| IBIS file stm32mp251_253_255_257_tfbga436.ibs
[IBIS ver] 5.1
[File name] stm32mp251_253_255_257_tfbga436.ibs
[File Rev] 1.3
[Date] 09-10-2025
[Source] Data Created at STMicroelectronics
[Notes]  File originated from ELDO simulations.
[Disclaimer]  This information is for modeling purpose only and is
   not guaranted. The information is subject to change without
   notice.
[Copyright] Copyright 2025 STMicroelectronics Inc.
|   Component stm32mp251_253_255_257_tfbga436
[Component] stm32mp251_253_255_257_tfbga436
[Manufacturer] STMicroelectronics
[Package]
| variable   typ   min   max
R_pkg   0.0   0.0   0.0
L_pkg   0.0H   0.0H   0.0H
C_pkg   0.0F   0.0F   0.0F
[Pin]  signal_name   model_name   R_pin   L_pin   C_pin
A1  VSS  gnd
A2  LVDS2_D1P  nc
A3  LVDS2_D1N  nc
A4  LVDS2_D0P  nc
A7  DSI_D3P  DPHY_IBIS
A8  DSI_CKP  DPHY_IBIS
A11  PB10  io8_tt
A12  PB9  io8_tt
A15  PD6  io8_tt
A16  PE0  io8_tt
A19  PE10  io8_tt
A20  PE14  io8_tt
A21  PD12  io8_tt
A22  VSS  gnd
AA1  JTCK_SWCLK  io8_tt
AA2  NJTRST  io8_tt
AA3  PJ3  io8_tt
AA4  PG4  io8_tt
AA6  PF10  io8_tt
AA7  PF9  io8_tt
AA8  PF8  io8_tt
AA10  PC6  io8_tt_i3c
AA11  PH12  io8_tt
AA12  PC0  io8_tt
AA14  PH6  io8_tt_i3c
AA15  PH5  io8_tt
AA16  USBH_HS_DP  USB2_HS_IBIS
AA18  PCIE_CLKINN  nc
AA19  COMBOPHY_TX1P  synopsys_usb3_tx
AA20  COMBOPHY_RX1P  synopsys_usb3_rx
AA21  PCIE_CLKOUTP  nc
AA22  DDR_DQ3  mal4drv27_PAD
AB1  VSS  gnd
AB2  JTDI  io8_tt
AB3  PJ2  io8_tt
AB4  PB15  io8_tt
AB7  PC11  io8_tt
AB8  PF6  io8_tt
AB11  PH13  io8_tt
AB12  PH9  io8_tt
AB15  PH4  io8_tt
AB16  USBH_HS_DM  USB2_HS_IBIS
AB19  COMBOPHY_TX1N  synopsys_usb3_tx
AB20  COMBOPHY_RX1N  synopsys_usb3_rx
AB21  PCIE_CLKOUTN  nc
AB22  VSS  gnd
B1  LVDS2_D4P  nc
B2  LVDS2_D4N  nc
B3  LVDS2_D2N  nc
B4  LVDS2_D0N  nc
B5  CSI_D0N  DPHY_IBIS_L1
B7  DSI_D3N  DPHY_IBIS
B8  DSI_CKN  DPHY_IBIS
B9  DSI_D0N  DPHY_IBIS
B11  PB5  io8_tt_i3c
B12  PB11  io8_tt
B13  PD9  io8_tt
B15  PD5  io8_tt
B16  PE1  io8_tt
B17  PE4  io8_tt
B19  PE13  io8_tt
B20  PB12  io8_tt
B21  PD13  io8_tt
B22  DDR_DQ19  mal4drv27_PAD
C1  LVDS2_D3P  nc
C2  LVDS2_D3N  nc
C3  LVDS2_D2P  nc
C4  VDDA18LVDS  power
C5  CSI_D0P  DPHY_IBIS_L1
C6  CSI_CKP  DPHY_IBIS_L1
C7  VDDA18DSI  power
C8  DSI_D2P  DPHY_IBIS
C9  DSI_D0P  DPHY_IBIS
C10  PB2  io8_tt
C11  PB0  io8_tt
C12  PB6  io8_tt
C13  PD8  io8_tt
C14  PD4  io8_tt
C15  PD3  io8_tt
C16  PE2  io8_tt
C17  PE5  io8_tt
C18  PE8  io8_tt
C19  PE12  io8_tt
C20  PB14  io8_tt
C21  DDR_DQ18  mal4drv27_PAD
C22  DDR_DQ17  mal4drv27_PAD
D1  LVDS1_D1N  nc
D2  LVDS1_D1P  nc
D3  LVDS1_D0N  nc
D4  LVDS1_D0P  nc
D5  VDDCSI  nc
D6  CSI_CKN  DPHY_IBIS_L1
D7  CSI_D1P  DPHY_IBIS_L1
D8  DSI_D2N  DPHY_IBIS
D9  DSI_D1P  DPHY_IBIS
D10  PB4  io8_tt_i3c
D11  PB1  io8_tt
D12  PB7  io8_tt
D13  PD10  io8_tt_i3c
D14  PD0  io8_tt
D15  PD7  io8_tt
D16  PE3  io8_tt
D17  PE7  io8_tt
D18  PE9  io8_tt
D19  PB13  io8_tt
D20  DDR_DQ16  mal4drv27_PAD
D21  DDR_DQS2P  mal4drv27_PAD
D22  DDR_DQS2N  mal4drv27_PAD
E3  LVDS1_D2P  nc
E4  LVDS1_D2N  nc
E5  VSS  gnd
E6  CSI_REXT  nc
E7  CSI_D1N  DPHY_IBIS_L1
E8  DSI_REXT  nc
E9  DSI_D1N  DPHY_IBIS
E10  PB3  io8_tt
E11  PI15  io8_tt
E12  PK1  io8_tt
E13  PD11  io8_tt_i3c
E14  PD2  io8_tt
E15  PD1  io8_tt
E16  PE6  io8_tt
E17  PE11  io8_tt
E18  PI11  io8_tt
E19  DDR_DQ22  mal4drv27_PAD
E20  DDR_DQ23  mal4drv27_PAD
E21  DDR_DQM2  mal4drv27_PAD
F2  LVDS1_D3P  nc
F3  LVDS1_D3N  nc
F4  LVDS1_D4P  nc
F5  LVDS1_D4N  nc
F6  VDDA18CSI  power
F7  VDDDSI  nc
F8  VDDIO3  power
F9  VDDIO3  power
F10  VDDIO2  power
F11  PK4  io8_tt
F12  PK0  io8_tt
F13  PK2  io8_tt_i3c
F14  PK5  io8_tt_i3c
F15  PK3  io8_tt
F16  PD15  io8_tt_i3c
F17  PE15  io8_tt
F18  DDR_RESETN  nc
F19  DDR_DQ21  mal4drv27_PAD
F20  DDR_DQ20  mal4drv27_PAD
G1  PI12  io8_tt
G2  PI13  io8_tt
G3  PG9  io8_tt
G4  PG14  io8_tt
G5  PI0  io8_tt
G6  VSS  gnd
G7  VDDLVDS  nc
G8  VDDIO4  power
G9  VDDIO4  power
G10  VDDIO1  power
G11  PB8  io8_tt
G12  PK6  io8_tt_i3c
G13  PI14  io8_tt
G14  PK7  io8_tt_i3c
G15  PD14  io8_tt_i3c
G16  PI10  io8_tt
G17  VDDA18PLL1  nc
G18  DDR_A20  mal4drv20_PAD
G19  DDR_DQ24  mal4drv27_PAD
G20  DDR_DQ27  mal4drv27_PAD
G21  DDR_DQ26  mal4drv27_PAD
G22  DDR_DQ25  mal4drv27_PAD
H1  PF14  io8_tt
H2  PG6  io8_tt_i3c
H3  PG10  io8_tt
H4  PG15  io8_tt
H5  PI5  io8_tt
H6  PI1  io8_tt_i3c
H7  VDDCORE  nc
H8  VSS  gnd
H9  VDDCORE  nc
H10  VSS  gnd
H11  VDDCPU  nc
H12  VSS  gnd
H13  VDDCPU  nc
H14  VSS  gnd
H15  VDDCPU  nc
H16  VSS  gnd
H17  DDR_A22  mal4drv20_PAD
H18  DDR_A17  mal4drv20_PAD
H19  DDR_A18  mal4drv20_PAD
H20  DDR_DQM3  mal4drv27_PAD
H21  DDR_DQS3N  mal4drv27_PAD
H22  DDR_DQS3P  mal4drv27_PAD
J3  PG12  io8_tt
J4  PG11  io8_tt
J5  PI2  io8_tt
J6  PI3  io8_tt
J7  PI6  io8_tt
J8  VDDCORE  nc
J9  VSS  gnd
J10  VDDCORE  nc
J11  VSS  gnd
J12  VDDCPU  nc
J13  VSS  gnd
J14  VDDCPU  nc
J15  VSS  gnd
J16  VDDA18DDR  nc
J17  DDR_A23  mal4drv20_PAD
J18  DDR_A16  mal4drv20_PAD
J19  DDR_A21  mal4drv20_PAD
J20  DDR_DQ29  mal4drv27_PAD
J21  DDR_DQ28  mal4drv27_PAD
K2  PJ15  io8_tt
K3  PF12  io8_tt
K4  PG7  io8_tt
K5  PG13  io8_tt_i3c
K6  PI4  io8_tt
K7  PI9  io8_tt
K8  VDDA18PLL2  nc
K9  VDDCORE  nc
K10  VSS  gnd
K11  VDDCORE  nc
K12  VSS  gnd
K13  VDDCPU  nc
K14  VSS  gnd
K15  VDDQDDR  power
K16  DDR_ZQ  nc
K17  DDR_A19  mal4drv20_PAD
K18  DDR_A13  mal4drv20_PAD
K19  DDR_A12  mal4drv20_PAD
K20  DDR_DQ30  mal4drv27_PAD
L1  PG5  io8_tt_i3c
L2  PJ12  io8_tt_i3c
L3  PJ14  io8_tt
L4  PF13  io8_tt
L5  PG8  io8_tt
L6  PI7  io8_tt
L7  PF15  io8_tt
L8  VDDA18PLL3  nc
L9  VSS  gnd
L10  VDDCORE  nc
L11  VSS  gnd
L12  VDDCPU  nc
L13  VSS  gnd
L14  VDDQDDR  power
L15  VSS  gnd
L16  VDDQDDR  power
L17  DDR_A15  mal4drv20_PAD
L18  DDR_A14  mal4drv20_PAD
L19  DDR_DQ31  mal4drv27_PAD
L20  DDR_VREF  nc
L21  DDR_DQ10  mal4drv27_PAD
L22  DDR_DQ11  mal4drv27_PAD
M1  PJ9  io8_tt
M2  PJ8  io8_tt
M3  PJ10  io8_tt_i3c
M4  PJ13  io8_tt_i3c
M5  PJ11  io8_tt
M6  PI8  io8_tt
M7  VSSAON  gnd
M8  V08CAP  nc
M9  VDD  power
M10  VSS  gnd
M11  VDDGPU  nc
M12  VSS  gnd
M13  VDDGPU  nc
M14  VSS  gnd
M15  VDDQDDR  power
M16  DDR_A0  mal4drv20_PAD
M17  DDR_A3  mal4drv20_PAD
M18  DDR_A28  mal4drv20_PAD
M19  DDR_A5  mal4drv20_PAD
M20  VSS  gnd
M21  DDR_DQ8  mal4drv27_PAD
M22  DDR_DQ9  mal4drv27_PAD
N3  PZ9  io8_tt_i3c
N4  PZ3  io8_tt_i3c
N5  PZ0  io8_tt_i3c
N6  PZ1  io8_tt_i3c
N7  VSS  gnd
N8  VDD  power
N9  VSS  gnd
N10  VDDGPU  nc
N11  VSS  gnd
N12  VDDGPU  nc
N13  VSS  gnd
N14  VDDQDDR  power
N15  VSS  gnd
N16  DDR_A2  mal4drv20_PAD
N17  DDR_A11  mal4drv20_PAD
N18  DDR_A10  mal4drv20_PAD
N19  DDR_A4  mal4drv20_PAD
N20  DDR_DQS1P  mal4drv27_PAD
N21  DDR_DQS1N  mal4drv27_PAD
P2  PZ7  io8_tt
P3  PZ8  io8_tt
P4  PZ2  io8_tt_i3c
P5  PZ5  io8_tt
P6  PC13  io8_tt
P7  VBAT  power
P8  VSS  gnd
P9  VDD  power
P10  VSS  gnd
P11  VDD  power
P12  VSS  gnd
P13  VDDGPU  nc
P14  VSS  gnd
P15  VDDQDDR  power
P16  DDR_A31  mal4drv20_PAD
P17  DDR_A30  mal4drv20_PAD
P18  DDR_A9  mal4drv20_PAD
P19  DDR_A8  mal4drv20_PAD
P20  DDR_DQM1  mal4drv27_PAD
R1  OSC32_IN  isudq_tt
R2  OSC32_OUT  isudq_tt
R3  BOOT1  isudq_tt
R4  BOOT0  isudq_tt
R5  PZ4  io8_tt_i3c
R6  PZ6  io8_tt
R7  VDDA18AON  power
R8  VDD  power
R9  VSS  gnd
R10  VDD  power
R11  VSS  gnd
R12  VDDGPU  nc
R13  VSS  gnd
R14  VDDQDDR  power
R15  VSS  gnd
R16  VDDQDDR  power
R17  DDR_A25  mal4drv20_PAD
R18  DDR_A27  mal4drv20_PAD
R19  DDR_A26  mal4drv20_PAD
R20  DDR_DQ13  mal4drv27_PAD
R21  DDR_DQ14  mal4drv27_PAD
R22  DDR_DQ15  mal4drv27_PAD
T1  BOOT3  isudq_tt
T2  BOOT2  isudq_tt
T3  NRSTC1MS  io8_tt
T4  VSS  gnd
T5  PWR_ON  io8_tt
T6  PWR_CPUON  io8_tt
T7  PDR_ON  nc
T8  PC10  io8_tt
T9  PF7  io8_tt
T10  PA15  io8_tt_i3c
T11  PH11  io8_tt
T12  PA9  io8_tt
T13  PH7  io8_tt_i3c
T14  PA3  io8_tt_i3c
T15  UCPD1_CC1  nc
T16  VDD33UCPD  nc
T17  UCPD1_CC2  nc
T18  DDR_A6  mal4drv20_PAD
T19  DDR_A29  mal4drv20_PAD
T20  DDR_DQ5  mal4drv27_PAD
T21  DDR_DQ4  mal4drv27_PAD
T22  DDR_DQ12  mal4drv27_PAD
U3  NRST  nc
U4  PWR_LP  io8_tt
U5  PJ6  io8_tt
U6  VSS  gnd
U7  VSSA  nc
U8  PC9  io8_tt
U9  PC5  io8_tt_i3c
U10  PA14  io8_tt
U11  PH10  io8_tt
U12  PA12  io8_tt_i3c
U13  PA10  io8_tt
U14  PH8  io8_tt
U15  PJ0  io8_tt
U16  USB3DR_VBUS  nc
U17  VDDA18USB  power
U18  DDR_A1  mal4drv20_PAD
U19  DDR_A7  mal4drv20_PAD
U20  DDR_DQ7  mal4drv27_PAD
U21  DDR_DQ6  mal4drv27_PAD
V2  OSC_OUT  isudq_tt
V3  OSC_IN  isudq_tt
V4  PJ5  io8_tt
V5  ANA0  nc
V6  ANA1  nc
V7  VDDA18ADC  power
V8  PC8  io8_tt
V9  PC4  io8_tt
V10  PF2  io8_tt_i3c
V11  PC1  io8_tt_i3c
V12  PF0  io8_tt_i3c
V13  PH2  io8_tt_i3c
V14  PA6  io8_tt
V15  PA1  io8_tt_i3c
V16  USBH_HS_TXRTUNE  nc
V17  USB3DR_TXRTUNE  nc
V18  VDDPCIECLK  nc
V19  VDDCOMBOPHY  nc
V20  DDR_DQS0P  mal4drv27_PAD
W1  JTDO_TRACESWO  io8_tt
W2  PJ7  io8_tt
W3  PJ4  io8_tt
W4  PG3  io8_tt
W5  VREFN  nc
W6  PG1  io8_tt_i3c
W7  PG0  io8_tt_i3c
W8  VSS  gnd
W9  PC3  io8_tt
W10  PF3  io8_tt
W11  PF1  io8_tt
W12  PA11  io8_tt
W13  PA2  io8_tt_i3c
W14  PH3  io8_tt_i3c
W15  PA8  io8_tt_i3c
W16  VSS  gnd
W17  USB3DR_DP  USB2_HS_IBIS
W18  VDDA18COMBOPHY  power
W19  VSS  gnd
W20  DDR_DQS0N  mal4drv27_PAD
W21  DDR_DQM0  mal4drv27_PAD
W22  DDR_DQ0  mal4drv27_PAD
Y1  JTMS_SWDIO  io8_tt
Y2  PA0  io8_tt
Y3  PJ1  io8_tt_i3c
Y4  PG2  io8_tt_i3c
Y5  VREFP  nc
Y6  PF11  io8_tt
Y7  PC12  io8_tt_i3c
Y8  PC7  io8_tt
Y9  PF5  io8_tt
Y10  PF4  io8_tt
Y11  PC2  io8_tt
Y12  PA13  io8_tt
Y13  PA5  io8_tt
Y14  PA7  io8_tt
Y15  PA4  io8_tt
Y16  VDD33USB  power
Y17  USB3DR_DM  USB2_HS_IBIS
Y18  PCIE_CLKINP  nc
Y19  VDDCOMBOPHYTX  nc
Y20  COMBOPHY_REXT  nc
Y21  DDR_DQ1  mal4drv27_PAD
Y22  DDR_DQ2  mal4drv27_PAD
[Package Model]   505-fcbga-18x18-436-240122
[Pin Mapping]   pulldown_ref   pullup_ref   | Comment
A1  gnd  nc
A2  nc  nc
A3  nc  nc
A4  nc  nc
A7  gnd  VDDA18DSI
A8  gnd  VDDA18DSI
A11  gnd  vddio4
A12  gnd  vddio4
A15  gnd  vddio3
A16  gnd  vddio1
A19  gnd  vddio2
A20  gnd  vddio2
A21  gnd  vdd
A22  gnd  nc
AA1  gnd  vdd
AA2  gnd  vdd
AA3  gnd  vdd
AA4  gnd  vdd
AA6  gnd  vdd
AA7  gnd  vdd
AA8  gnd  vdd
AA10  gnd  vdd
AA11  gnd  vdd
AA12  gnd  vdd
AA14  gnd  vdd
AA15  gnd  vdd
AA16  gnd  VDD33USB
AA18  nc  nc
AA19  gnd  VDDA18COMBOPHY
AA20  gnd  VDDA18COMBOPHY
AA21  nc  nc
AA22  gnd  vddqddr
AB1  gnd  nc
AB2  gnd  vdd
AB3  gnd  vdd
AB4  gnd  vdd
AB7  gnd  vdd
AB8  gnd  vdd  | Depending on IO usage
| AB8  gnd  vsw  | Depending on IO usage
AB11  gnd  vdd
AB12  gnd  vdd
AB15  gnd  vdd
AB16  gnd  VDD33USB
AB19  gnd  VDDA18COMBOPHY
AB20  gnd  VDDA18COMBOPHY
AB21  nc  nc
AB22  gnd  nc
B1  nc  nc
B2  nc  nc
B3  nc  nc
B4  nc  nc
B5  gnd  VDDA18CSI
B7  gnd  VDDA18DSI
B8  gnd  VDDA18DSI
B9  gnd  VDDA18DSI
B11  gnd  vddio4
B12  gnd  vddio4
B13  gnd  vddio3
B15  gnd  vddio3
B16  gnd  vddio1
B17  gnd  vddio1
B19  gnd  vddio2
B20  gnd  vdd
B21  gnd  vdd
B22  gnd  vddqddr
C1  nc  nc
C2  nc  nc
C3  nc  nc
C4  nc  vdda18lvds
C5  gnd  VDDA18CSI
C6  gnd  VDDA18CSI
C7  nc  VDDA18DSI
C8  gnd  VDDA18DSI
C9  gnd  VDDA18DSI
C10  gnd  vddio4
C11  gnd  vddio4
C12  gnd  vddio4
C13  gnd  vddio3
C14  gnd  vddio3
C15  gnd  vddio3
C16  gnd  vddio1
C17  gnd  vddio1
C18  gnd  vddio2
C19  gnd  vddio2
C20  gnd  vdd
C21  gnd  vddqddr
C22  gnd  vddqddr
D1  nc  nc
D2  nc  nc
D3  nc  nc
D4  nc  nc
D5  nc  nc
D6  gnd  VDDA18CSI
D7  gnd  VDDA18CSI
D8  gnd  VDDA18DSI
D9  gnd  VDDA18DSI
D10  gnd  vddio4
D11  gnd  vddio4
D12  gnd  vddio4
D13  gnd  vddio3
D14  gnd  vddio3
D15  gnd  vddio3
D16  gnd  vddio1
D17  gnd  vddio2
D18  gnd  vddio2
D19  gnd  vdd
D20  gnd  vddqddr
D21  gnd  vddqddr
D22  gnd  vddqddr
E3  nc  nc
E4  nc  nc
E5  gnd  nc
E6  nc  nc
E7  gnd  VDDA18CSI
E8  nc  nc
E9  gnd  VDDA18DSI
E10  gnd  vddio4
E11  gnd  vdd
E12  gnd  vdd
E13  gnd  vddio3
E14  gnd  vddio3
E15  gnd  vddio3
E16  gnd  vddio2
E17  gnd  vddio2
E18  gnd  vdd
E19  gnd  vddqddr
E20  gnd  vddqddr
E21  gnd  vddqddr
F2  nc  nc
F3  nc  nc
F4  nc  nc
F5  nc  nc
F6  nc  VDDA18CSI
F7  nc  nc
F8  nc  vddio3
F9  nc  vddio3
F10  nc  vddio2
F11  gnd  vdd
F12  gnd  vdd
F13  gnd  vdd
F14  gnd  vdd
F15  gnd  vdd
F16  gnd  vdd
F17  gnd  vddio2
F18  nc  nc
F19  gnd  vddqddr
F20  gnd  vddqddr
G1  gnd  vdd
G2  gnd  vdd
G3  gnd  vdd
G4  gnd  vdd
G5  gnd  vdd
G6  gnd  nc
G7  nc  nc
G8  nc  vddio4
G9  nc  vddio4
G10  nc  vddio1
G11  gnd  vddio4
G12  gnd  vdd
G13  gnd  vdd
G14  gnd  vdd
G15  gnd  vdd
G16  gnd  vdd
G17  nc  nc
G18  gnd  vddqddr
G19  gnd  vddqddr
G20  gnd  vddqddr
G21  gnd  vddqddr
G22  gnd  vddqddr
H1  gnd  vdd
H2  gnd  vdd
H3  gnd  vdd
H4  gnd  vdd
H5  gnd  vdd
H6  gnd  vdd
H7  nc  nc
H8  gnd  nc
H9  nc  nc
H10  gnd  nc
H11  nc  nc
H12  gnd  nc
H13  nc  nc
H14  gnd  nc
H15  nc  nc
H16  gnd  nc
H17  gnd  vddqddr
H18  gnd  vddqddr
H19  gnd  vddqddr
H20  gnd  vddqddr
H21  gnd  vddqddr
H22  gnd  vddqddr
J3  gnd  vdd
J4  gnd  vdd
J5  gnd  vdd
J6  gnd  vdd
J7  gnd  vdd
J8  nc  nc
J9  gnd  nc
J10  nc  nc
J11  gnd  nc
J12  nc  nc
J13  gnd  nc
J14  nc  nc
J15  gnd  nc
J16  nc  nc
J17  gnd  vddqddr
J18  gnd  vddqddr
J19  gnd  vddqddr
J20  gnd  vddqddr
J21  gnd  vddqddr
K2  gnd  vdd
K3  gnd  vdd
K4  gnd  vdd
K5  gnd  vdd
K6  gnd  vdd
K7  gnd  vdd
K8  nc  nc
K9  nc  nc
K10  gnd  nc
K11  nc  nc
K12  gnd  nc
K13  nc  nc
K14  gnd  nc
K15  nc  vddqddr
K16  nc  nc
K17  gnd  vddqddr
K18  gnd  vddqddr
K19  gnd  vddqddr
K20  gnd  vddqddr
L1  gnd  vdd
L2  gnd  vdd
L3  gnd  vdd
L4  gnd  vdd
L5  gnd  vdd
L6  gnd  vdd
L7  gnd  vdd
L8  nc  nc
L9  gnd  nc
L10  nc  nc
L11  gnd  nc
L12  nc  nc
L13  gnd  nc
L14  nc  vddqddr
L15  gnd  nc
L16  nc  vddqddr
L17  gnd  vddqddr
L18  gnd  vddqddr
L19  gnd  vddqddr
L20  nc  nc
L21  gnd  vddqddr
L22  gnd  vddqddr
M1  gnd  vdd
M2  gnd  vdd
M3  gnd  vdd
M4  gnd  vdd
M5  gnd  vdd
M6  gnd  vdd  | Depending on IO usage
| M6  gnd  vsw  | Depending on IO usage
M7  gnd_aon  nc
M8  nc  nc
M9  nc  vdd
M10  gnd  nc
M11  nc  nc
M12  gnd  nc
M13  nc  nc
M14  gnd  nc
M15  nc  vddqddr
M16  gnd  vddqddr
M17  gnd  vddqddr
M18  gnd  vddqddr
M19  gnd  vddqddr
M20  gnd  nc
M21  gnd  vddqddr
M22  gnd  vddqddr
N3  gnd  vdd
N4  gnd  vdd  | Depending on IO usage
| N4  gnd  vsw  | Depending on IO usage
N5  gnd  vdd  | Depending on IO usage
| N5  gnd  vsw  | Depending on IO usage
N6  gnd  vdd  | Depending on IO usage
| N6  gnd  vsw  | Depending on IO usage
N7  gnd  nc
N8  nc  vdd
N9  gnd  nc
N10  nc  nc
N11  gnd  nc
N12  nc  nc
N13  gnd  nc
N14  nc  vddqddr
N15  gnd  nc
N16  gnd  vddqddr
N17  gnd  vddqddr
N18  gnd  vddqddr
N19  gnd  vddqddr
N20  gnd  vddqddr
N21  gnd  vddqddr
P2  gnd  vdd
P3  gnd  vdd
P4  gnd  vdd  | Depending on IO usage
| P4  gnd  vsw  | Depending on IO usage
P5  gnd  vdd  | Depending on IO usage
| P5  gnd  vsw  | Depending on IO usage
P6  gnd  vdd  | Depending on IO usage
| P6  gnd  vsw  | Depending on IO usage
P7  nc  vsw
P8  gnd  nc
P9  nc  vdd
P10  gnd  nc
P11  nc  vdd
P12  gnd  nc
P13  nc  nc
P14  gnd  nc
P15  nc  vddqddr
P16  gnd  vddqddr
P17  gnd  vddqddr
P18  gnd  vddqddr
P19  gnd  vddqddr
P20  gnd  vddqddr
R1  gnd  vdd  | Depending on IO usage
| R1  gnd  vsw  | Depending on IO usage
R2  gnd  vdd  | Depending on IO usage
| R2  gnd  vsw  | Depending on IO usage
R3  gnd  vdd
R4  gnd  vdd
R5  gnd  vdd  | Depending on IO usage
| R5  gnd  vsw  | Depending on IO usage
R6  gnd  vdd  | Depending on IO usage
| R6  gnd  vsw  | Depending on IO usage
R7  nc  vdda18aon
R8  nc  vdd
R9  gnd  nc
R10  nc  vdd
R11  gnd  nc
R12  nc  nc
R13  gnd  nc
R14  nc  vddqddr
R15  gnd  nc
R16  nc  vddqddr
R17  gnd  vddqddr
R18  gnd  vddqddr
R19  gnd  vddqddr
R20  gnd  vddqddr
R21  gnd  vddqddr
R22  gnd  vddqddr
T1  gnd  vdd
T2  gnd  vdd
T3  gnd  vdd
T4  gnd  nc
T5  gnd  vdd
T6  gnd  vdd
T7  nc  nc
T8  gnd  vdd
T9  gnd  vdd  | Depending on IO usage
| T9  gnd  vsw  | Depending on IO usage
T10  gnd  vdd
T11  gnd  vdd
T12  gnd  vdd
T13  gnd  vdd
T14  gnd  vdd
T15  nc  nc
T16  nc  nc
T17  nc  nc
T18  gnd  vddqddr
T19  gnd  vddqddr
T20  gnd  vddqddr
T21  gnd  vddqddr
T22  gnd  vddqddr
U3  nc  nc
U4  gnd  vdd
U5  gnd  vdd
U6  gnd  nc
U7  nc  nc
U8  gnd  vdd
U9  gnd  vdd  | Depending on IO usage
| U9  gnd  vsw  | Depending on IO usage
U10  gnd  vdd
U11  gnd  vdd
U12  gnd  vdd
U13  gnd  vdd
U14  gnd  vdd
U15  gnd  vdd
U16  nc  nc
U17  nc  vdda18usb
U18  gnd  vddqddr
U19  gnd  vddqddr
U20  gnd  vddqddr
U21  gnd  vddqddr
V2  gnd_aon  vdda18aon
V3  gnd_aon  vdda18aon
V4  gnd  vdd
V5  nc  nc
V6  nc  nc
V7  nc  vdda18adc
V8  gnd  vdd
V9  gnd  vdd  | Depending on IO usage
| V9  gnd  vsw  | Depending on IO usage
V10  gnd  vdd
V11  gnd  vdd
V12  gnd  vdd
V13  gnd  vdd
V14  gnd  vdd
V15  gnd  vdd
V16  nc  nc
V17  nc  nc
V18  nc  nc
V19  nc  nc
V20  gnd  vddqddr
W1  gnd  vdd
W2  gnd  vdd
W3  gnd  vdd
W4  gnd  vdd  | Depending on IO usage
| W4  gnd  vsw  | Depending on IO usage
W5  nc  nc
W6  gnd  vdd  | Depending on IO usage
| W6  gnd  vsw  | Depending on IO usage
W7  gnd  vdd
W8  gnd  nc
W9  gnd  vdd  | Depending on IO usage
| W9  gnd  vsw  | Depending on IO usage
W10  gnd  vdd
W11  gnd  vdd
W12  gnd  vdd
W13  gnd  vdd
W14  gnd  vdd
W15  gnd  vdd
W16  gnd  nc
W17  gnd  VDD33USB
W18  nc  VDDA18COMBOPHY
W19  gnd  nc
W20  gnd  vddqddr
W21  gnd  vddqddr
W22  gnd  vddqddr
Y1  gnd  vdd
Y2  gnd  vdd
Y3  gnd  vdd
Y4  gnd  vdd
Y5  nc  nc
Y6  gnd  vdd
Y7  gnd  vdd
Y8  gnd  vdd
Y9  gnd  vdd
Y10  gnd  vdd
Y11  gnd  vdd
Y12  gnd  vdd
Y13  gnd  vdd
Y14  gnd  vdd
Y15  gnd  vdd
Y16  nc  VDD33USB
Y17  gnd  VDD33USB
Y18  nc  nc
Y19  nc  nc
Y20  nc  nc
Y21  gnd  vddqddr
Y22  gnd  vddqddr
[Diff Pin]   inv_pin   vdiff   tdelay_typ   tdelay_min   tdelay_max
N19   M19   0.320V   0ns   NA   NA   |CKA
|J18   H18   0.320V   0ns   NA   NA   |CKB only in LPDDR4 32 bit
V20   W20   0.320V   0ns   NA   NA   |DQS0
N20   N21   0.320V   0ns   NA   NA   |DQS1
D21   D22   0.320V   0ns   NA   NA   |DQS2
H22   H21   0.320V   0ns   NA   NA   |DQS3
AA20   AB20   NA   NA   NA   NA
AA19   AB19   NA   NA   NA   NA
C6   D6   NA   NA   NA   NA
C5   B5   NA   NA   NA   NA
D7   E7   NA   NA   NA   NA
A8   B8   NA   NA   NA   NA  |DSI CKP CKN
C9   B9   400.000mV   0ns   NA   NA   |D0P D0N
D9   E9   400.000mV   0ns   NA   NA   |D1P D1N
C8   D8   400.000mV   0ns   NA   NA   |D2P D2N
A7   B7   400.000mV   0ns   NA   NA   |D3P D3N
D4   D3   NA   NA   NA   NA
D2   D1   NA   NA   NA   NA
E3   E4   NA   NA   NA   NA
F2   F3   NA   NA   NA   NA
F4   F5   NA   NA   NA   NA
A4   B4   NA   NA   NA   NA
A2   A3   NA   NA   NA   NA
C3   B3   NA   NA   NA   NA
C1   C2   NA   NA   NA   NA
B1   B2   NA   NA   NA   NA
Y18   AA18   NA   NA   NA   NA
AA21   AB21   NA   NA   NA   NA
W17   Y17   NA   NA   NA   NA   |USB3DR_DP _DM
AA16   AB16   NA   NA   NA   NA   |USBH_HS_DP _DM
[Model Selector] DPHY_IBIS_L1
DPHY_RX_2P5G_L1   DPHY HSRX model at 2.5Gbps for lane 1
DPHY_RX_1P5G_L1   DPHY HSRX model at 1.5Gbps for lane 1
[Model Selector] DPHY_IBIS
DPHY_TX_2P5G   DPHY HSTX model at 2.5Gbps
DPHY_TX_1P5G   DPHY HSTX model at 1.5Gbps
[Model Selector] USB2_HS_IBIS
USB2_HSRX   USB2 HSRX model
USB2_HSTX_00_0_01_0011_11   TuningBits_AMP_PULSE_RISE_REF_XV=00_0_01_0011_11
USB2_HSTX_00_0_10_0101_11   TuningBits_AMP_PULSE_RISE_REF_XV=00_0_10_0101_11
USB2_HSTX_00_0_11_0111_11   TuningBits_AMP_PULSE_RISE_REF_XV=00_0_11_0111_11
USB2_HSTX_00_1_01_0011_11   TuningBits_AMP_PULSE_RISE_REF_XV=00_1_01_0011_11
USB2_HSTX_00_1_10_0101_11   TuningBits_AMP_PULSE_RISE_REF_XV=00_1_10_0101_11
USB2_HSTX_00_1_11_0111_11   TuningBits_AMP_PULSE_RISE_REF_XV=00_1_11_0111_11
USB2_HSTX_01_0_01_0011_11   TuningBits_AMP_PULSE_RISE_REF_XV=01_0_01_0011_11
USB2_HSTX_01_0_10_0101_11   TuningBits_AMP_PULSE_RISE_REF_XV=01_0_10_0101_11
USB2_HSTX_01_0_11_0111_11   TuningBits_AMP_PULSE_RISE_REF_XV=01_0_11_0111_11
USB2_HSTX_01_1_01_0011_11   TuningBits_AMP_PULSE_RISE_REF_XV=01_1_01_0011_11
USB2_HSTX_01_1_10_0101_11   TuningBits_AMP_PULSE_RISE_REF_XV=01_1_10_0101_11
USB2_HSTX_01_1_11_0111_11   TuningBits_AMP_PULSE_RISE_REF_XV=01_1_11_0111_11
USB2_HSTX_10_0_01_0011_11   TuningBits_AMP_PULSE_RISE_REF_XV=10_0_01_0011_11
USB2_HSTX_10_0_10_0101_11   TuningBits_AMP_PULSE_RISE_REF_XV=10_0_10_0101_11
USB2_HSTX_10_0_11_0111_11   TuningBits_AMP_PULSE_RISE_REF_XV=10_0_11_0111_11
USB2_HSTX_10_1_01_0011_11   TuningBits_AMP_PULSE_RISE_REF_XV=10_1_01_0011_11
USB2_HSTX_10_1_10_0101_11   TuningBits_AMP_PULSE_RISE_REF_XV=10_1_10_0101_11
USB2_HSTX_10_1_11_0111_11   TuningBits_AMP_PULSE_RISE_REF_XV=10_1_11_0111_11
[Model Selector] io8_tt
io8_tt_ls_3v3   "GPIO - 3V tolerant - 3.3V range - Low speed"
io8_tt_ms_3v3   "GPIO - 3V tolerant - 3.3V range - Med speed"
io8_tt_fs_3v3   "GPIO - 3V tolerant - 3.3V range - Fast speed"
io8_tt_hs_3v3   "GPIO - 3V tolerant - 3.3V range - High speed"
io8_tt_hslv_ls_1v8   "GPIO HSLV - 3V tolerant - 1.8V range - Low speed"
io8_tt_hslv_ms_1v8   "GPIO HSLV - 3V tolerant - 1.8V range - Med speed"
io8_tt_hslv_fs_1v8   "GPIO HSLV - 3V tolerant - 1.8V range - Fast speed"
io8_tt_hslv_hs_1v8   "GPIO HSLV - 3V tolerant - 1.8V range - High speed"
[Model Selector] io8_tt_i3c
io8_tt_ls_3v3   "GPIO - 3V tolerant - 3.3V range - Low speed"
io8_tt_ms_3v3   "GPIO - 3V tolerant - 3.3V range - Med speed"
io8_tt_fs_3v3   "GPIO - 3V tolerant - 3.3V range - Fast speed"
io8_tt_hs_3v3   "GPIO - 3V tolerant - 3.3V range - High speed"
io8_tt_hslv_ls_1v8   "GPIO HSLV - 3V tolerant - 1.8V range - Low speed"
io8_tt_hslv_ms_1v8   "GPIO HSLV - 3V tolerant - 1.8V range - Med speed"
io8_tt_hslv_fs_1v8   "GPIO HSLV - 3V tolerant - 1.8V range - Fast speed"
io8_tt_hslv_hs_1v8   "GPIO HSLV - 3V tolerant - 1.8V range - High speed"
io8_tt_i3c_3v3   "GPIO - 3V tolerant - 3.3V range - Open drain"
[Model Selector] isudq_tt
isudq_tt_1v8   "Input Buffer - 3V tolerant - 1.8V range"
isudq_tt_3v3   "Input Buffer - 3V tolerant - 3.3V range"
[Model Selector]   mal4drv20_PAD
mal4drv20_d3l_40   DDR3L mal4drv20 cell  Z0=40-Ohm Driver
mal4drv20_d3l_60   DDR3L mal4drv20 cell  Z0=60-Ohm Driver
mal4drv20_d3l_120   DDR3L mal4drv20 cell  Z0=120-Ohm Driver
mal4drv20_d3_20   DDR3 mal4drv20 cell  Z0=20-Ohm Driver
mal4drv20_d3_24   DDR3 mal4drv20 cell  Z0=24-Ohm Driver
mal4drv20_d3_30   DDR3 mal4drv20 cell  Z0=30-Ohm Driver
mal4drv20_d3_40   DDR3 mal4drv20 cell  Z0=40-Ohm Driver
mal4drv20_d3_60   DDR3 mal4drv20 cell  Z0=60-Ohm Driver
mal4drv20_d4_20   DDR4 mal4drv20 cell  Z0=20-Ohm Driver
mal4drv20_d4_24   DDR4 mal4drv20 cell  Z0=24-Ohm Driver
mal4drv20_d4_30   DDR4 mal4drv20 cell  Z0=30-Ohm Driver
mal4drv20_d4_40   DDR4 mal4drv20 cell  Z0=40-Ohm Driver
mal4drv20_d4_60   DDR4 mal4drv20 cell  Z0=60-Ohm Driver
mal4drv20_dl4_20   LPDDR4 mal4drv20 cell  Z0=20-Ohm Driver
mal4drv20_dl4_24   LPDDR4 mal4drv20 cell  Z0=24-Ohm Driver
mal4drv20_dl4_30   LPDDR4 mal4drv20 cell  Z0=30-Ohm Driver
mal4drv20_dl4_40   LPDDR4 mal4drv20 cell  Z0=40-Ohm Driver
mal4drv20_dl4_60   LPDDR4 mal4drv20 cell  Z0=60-Ohm Driver
[Model Selector]   mal4drv27_PAD
mal4drv27_d3l_40   DDR3L mal4drv27 cell  Z0=40-Ohm Driver
mal4drv27_d3l_48   DDR3L mal4drv27 cell  Z0=48-Ohm Driver
mal4drv27_d3l_60   DDR3L mal4drv27 cell  Z0=60-Ohm Driver
mal4drv27_d3l_80   DDR3L mal4drv27 cell  Z0=80-Ohm Driver
mal4drv27_d3l_120   DDR3L mal4drv27 cell  Z0=120-Ohm Driver
mal4drv27_d3l_240   DDR3L mal4drv27 cell  Z0=240-Ohm Driver
mal4drv27_d3l_odt120   DDR3L mal4drv27 cell 120-Ohm ODT Receiver
mal4drv27_d3l_odt60   DDR3L mal4drv27 cell 60-Ohm ODT Receiver
mal4drv27_d3l_odtoff   DDR3L mal4drv27 cell ODT OFF Receiver
mal4drv27_d3_28   DDR3 mal4drv27 cell  Z0=28-Ohm Driver
mal4drv27_d3_34   DDR3 mal4drv27 cell  Z0=34-Ohm Driver
mal4drv27_d3_40   DDR3 mal4drv27 cell  Z0=40-Ohm Driver
mal4drv27_d3_53   DDR3 mal4drv27 cell  Z0=53-Ohm Driver
mal4drv27_d3_odt120   DDR3 mal4drv27 cell 120-Ohm ODT Receiver
mal4drv27_d3_odt60   DDR3 mal4drv27 cell 60-Ohm ODT Receiver
mal4drv27_d4_28   DDR4 mal4drv27 cell  Z0=28-Ohm Driver
mal4drv27_d4_34   DDR4 mal4drv27 cell  Z0=34-Ohm Driver
mal4drv27_d4_40   DDR4 mal4drv27 cell  Z0=40-Ohm Driver
mal4drv27_d4_53   DDR4 mal4drv27 cell  Z0=53-Ohm Driver
mal4drv27_d4_odt120   DDR4 mal4drv27 cell 120-Ohm ODT Receiver
mal4drv27_d4_odt240   DDR4 mal4drv27 cell 240-Ohm ODT Receiver
mal4drv27_d4_odt48   DDR4 mal4drv27 cell 48-Ohm ODT Receiver
mal4drv27_d4_odt60   DDR4 mal4drv27 cell 60-Ohm ODT Receiver
mal4drv27_d4_odt80   DDR4 mal4drv27 cell 80-Ohm ODT Receiver
mal4drv27_dl4_28   LPDDR4 mal4drv27 cell  Z0=28-Ohm Driver
mal4drv27_dl4_34   LPDDR4 mal4drv27 cell  Z0=34-Ohm Driver
mal4drv27_dl4_40   LPDDR4 mal4drv27 cell  Z0=40-Ohm Driver
mal4drv27_dl4_53   LPDDR4 mal4drv27 cell  Z0=53-Ohm Driver
mal4drv27_dl4_odt48   LPDDR4 mal4drv27 cell 48-Ohm ODT Receiver
mal4drv27_dl4_odt60   LPDDR4 mal4drv27 cell 60-Ohm ODT Receiver
[Define Package Model]  505-fcbga-18x18-436-240122
[Manufacturer]  unknown
[OEM]  unknown
[Description]  unknown
[Number Of Pins]  362
[Pin Numbers]
| Pin Name Terminal   Net Name   Starting Node   Ending Node
V5 | ANA0
V6 | ANA1
R4 | BOOT0
R3 | BOOT1
T2 | BOOT2
T1 | BOOT3
Y20 | COMBOPHY_REXT
AB20 | COMBOPHY_RX1N
AA20 | COMBOPHY_RX1P
AB19 | COMBOPHY_TX1N
AA19 | COMBOPHY_TX1P
D6 | CSI_CKN
C6 | CSI_CKP
B5 | CSI_D0N
C5 | CSI_D0P
E7 | CSI_D1N
D7 | CSI_D1P
E6 | CSI_REXT
M16 | DDR_A0
U18 | DDR_A1
N16 | DDR_A2
M17 | DDR_A3
N19 | DDR_A4
M19 | DDR_A5
T18 | DDR_A6
U19 | DDR_A7
P19 | DDR_A8
P18 | DDR_A9
N18 | DDR_A10
N17 | DDR_A11
K19 | DDR_A12
K18 | DDR_A13
L18 | DDR_A14
L17 | DDR_A15
J18 | DDR_A16
H18 | DDR_A17
H19 | DDR_A18
K17 | DDR_A19
G18 | DDR_A20
J19 | DDR_A21
H17 | DDR_A22
J17 | DDR_A23
R17 | DDR_A25
R19 | DDR_A26
R18 | DDR_A27
M18 | DDR_A28
T19 | DDR_A29
P17 | DDR_A30
P16 | DDR_A31
W22 | DDR_DQ0
Y21 | DDR_DQ1
Y22 | DDR_DQ2
AA22 | DDR_DQ3
T21 | DDR_DQ4
T20 | DDR_DQ5
U21 | DDR_DQ6
U20 | DDR_DQ7
M21 | DDR_DQ8
M22 | DDR_DQ9
L21 | DDR_DQ10
L22 | DDR_DQ11
T22 | DDR_DQ12
R20 | DDR_DQ13
R21 | DDR_DQ14
R22 | DDR_DQ15
D20 | DDR_DQ16
C22 | DDR_DQ17
C21 | DDR_DQ18
B22 | DDR_DQ19
F20 | DDR_DQ20
F19 | DDR_DQ21
E19 | DDR_DQ22
E20 | DDR_DQ23
G19 | DDR_DQ24
G22 | DDR_DQ25
G21 | DDR_DQ26
G20 | DDR_DQ27
J21 | DDR_DQ28
J20 | DDR_DQ29
K20 | DDR_DQ30
L19 | DDR_DQ31
W21 | DDR_DQM0
P20 | DDR_DQM1
E21 | DDR_DQM2
H20 | DDR_DQM3
W20 | DDR_DQS0N
V20 | DDR_DQS0P
N21 | DDR_DQS1N
N20 | DDR_DQS1P
D22 | DDR_DQS2N
D21 | DDR_DQS2P
H21 | DDR_DQS3N
H22 | DDR_DQS3P
F18 | DDR_RESETN
L20 | DDR_VREF
K16 | DDR_ZQ
B8 | DSI_CKN
A8 | DSI_CKP
B9 | DSI_D0N
C9 | DSI_D0P
E9 | DSI_D1N
D9 | DSI_D1P
D8 | DSI_D2N
C8 | DSI_D2P
B7 | DSI_D3N
A7 | DSI_D3P
E8 | DSI_REXT
AA1 | JTCK_SWCLK
AB2 | JTDI
W1 | JTDO_TRACESWO
Y1 | JTMS_SWDIO
D3 | LVDS1_D0N
D4 | LVDS1_D0P
D1 | LVDS1_D1N
D2 | LVDS1_D1P
E4 | LVDS1_D2N
E3 | LVDS1_D2P
F3 | LVDS1_D3N
F2 | LVDS1_D3P
F5 | LVDS1_D4N
F4 | LVDS1_D4P
B4 | LVDS2_D0N
A4 | LVDS2_D0P
A3 | LVDS2_D1N
A2 | LVDS2_D1P
B3 | LVDS2_D2N
C3 | LVDS2_D2P
C2 | LVDS2_D3N
C1 | LVDS2_D3P
B2 | LVDS2_D4N
B1 | LVDS2_D4P
AA2 | NJTRST
U3 | NRST
T3 | NRSTC1MS
R1 | OSC32_IN
R2 | OSC32_OUT
V3 | OSC_IN
V2 | OSC_OUT
Y2 | PA0
V15 | PA1
W13 | PA2
T14 | PA3
Y15 | PA4
Y13 | PA5
V14 | PA6
Y14 | PA7
W15 | PA8
T12 | PA9
U13 | PA10
W12 | PA11
U12 | PA12
Y12 | PA13
U10 | PA14
T10 | PA15
C11 | PB0
D11 | PB1
C10 | PB2
E10 | PB3
D10 | PB4
B11 | PB5
C12 | PB6
D12 | PB7
G11 | PB8
A12 | PB9
A11 | PB10
B12 | PB11
B20 | PB12
D19 | PB13
C20 | PB14
AB4 | PB15
AA12 | PC0
V11 | PC1
Y11 | PC2
W9 | PC3
V9 | PC4
U9 | PC5
AA10 | PC6
Y8 | PC7
V8 | PC8
U8 | PC9
T8 | PC10
AB7 | PC11
Y7 | PC12
P6 | PC13
AA18 | PCIE_CLKINN
Y18 | PCIE_CLKINP
AB21 | PCIE_CLKOUTN
AA21 | PCIE_CLKOUTP
D14 | PD0
E15 | PD1
E14 | PD2
C15 | PD3
C14 | PD4
B15 | PD5
A15 | PD6
D15 | PD7
C13 | PD8
B13 | PD9
D13 | PD10
E13 | PD11
A21 | PD12
B21 | PD13
G15 | PD14
F16 | PD15
T7 | PDR_ON
A16 | PE0
B16 | PE1
C16 | PE2
D16 | PE3
B17 | PE4
C17 | PE5
E16 | PE6
D17 | PE7
C18 | PE8
D18 | PE9
A19 | PE10
E17 | PE11
C19 | PE12
B19 | PE13
A20 | PE14
F17 | PE15
V12 | PF0
W11 | PF1
V10 | PF2
W10 | PF3
Y10 | PF4
Y9 | PF5
AB8 | PF6
T9 | PF7
AA8 | PF8
AA7 | PF9
AA6 | PF10
Y6 | PF11
K3 | PF12
L4 | PF13
H1 | PF14
L7 | PF15
W7 | PG0
W6 | PG1
Y4 | PG2
W4 | PG3
AA4 | PG4
L1 | PG5
H2 | PG6
K4 | PG7
L5 | PG8
G3 | PG9
H3 | PG10
J4 | PG11
J3 | PG12
K5 | PG13
G4 | PG14
H4 | PG15
V13 | PH2
W14 | PH3
AB15 | PH4
AA15 | PH5
AA14 | PH6
T13 | PH7
U14 | PH8
AB12 | PH9
U11 | PH10
T11 | PH11
AA11 | PH12
AB11 | PH13
G5 | PI0
H6 | PI1
J5 | PI2
J6 | PI3
K6 | PI4
H5 | PI5
J7 | PI6
L6 | PI7
M6 | PI8
K7 | PI9
G16 | PI10
E18 | PI11
G1 | PI12
G2 | PI13
G13 | PI14
E11 | PI15
U15 | PJ0
Y3 | PJ1
AB3 | PJ2
AA3 | PJ3
W3 | PJ4
V4 | PJ5
U5 | PJ6
W2 | PJ7
M2 | PJ8
M1 | PJ9
M3 | PJ10
M5 | PJ11
L2 | PJ12
M4 | PJ13
L3 | PJ14
K2 | PJ15
F12 | PK0
E12 | PK1
F13 | PK2
F15 | PK3
F11 | PK4
F14 | PK5
G12 | PK6
G14 | PK7
T6 | PWR_CPUON
U4 | PWR_LP
T5 | PWR_ON
N5 | PZ0
N6 | PZ1
P4 | PZ2
N4 | PZ3
R5 | PZ4
P5 | PZ5
R6 | PZ6
P2 | PZ7
P3 | PZ8
N3 | PZ9
T15 | UCPD1_CC1
T17 | UCPD1_CC2
Y17 | USB3DR_DM
W17 | USB3DR_DP
V17 | USB3DR_TXRTUNE
U16 | USB3DR_VBUS
AB16 | USBH_HS_DM
AA16 | USBH_HS_DP
V16 | USBH_HS_TXRTUNE
M8 | V08CAP
P7 | VBAT
T16 | VDD33UCPD
Y16 | VDD33USB
M9 | VDD
V7 | VDDA18ADC
R7 | VDDA18AON
W18 | VDDA18COMBOPHY
F6 | VDDA18CSI
J16 | VDDA18DDR
C7 | VDDA18DSI
C4 | VDDA18LVDS
G17 | VDDA18PLL1
K8 | VDDA18PLL2
L8 | VDDA18PLL3
U17 | VDDA18USB
V19 | VDDCOMBOPHY
Y19 | VDDCOMBOPHYTX
H7 | VDDCORE
H11 | VDDCPU
D5 | VDDCSI
F7 | VDDDSI
M11 | VDDGPU
G10 | VDDIO1
F10 | VDDIO2
F8 | VDDIO3
G8 | VDDIO4
G7 | VDDLVDS
V18 | VDDPCIECLK
K15 | VDDQDDR
W5 | VREFN
Y5 | VREFP
A1 | VSS
U7 | VSSA
M7 | VSSAON
|[Merged Pins]  M9
|N8  |  VDD
|P9  |  VDD
|P11  |  VDD
|R8  |  VDD
|R10  |  VDD
|[Merged Pins]  H7
|H9  |  VDDCORE
|J8  |  VDDCORE
|J10  |  VDDCORE
|K9  |  VDDCORE
|K11  |  VDDCORE
|L10  |  VDDCORE
|[Merged Pins]  H11
|H13  |  VDDCPU
|H15  |  VDDCPU
|J12  |  VDDCPU
|J14  |  VDDCPU
|K13  |  VDDCPU
|L12  |  VDDCPU
|[Merged Pins]  M11
|M13  |  VDDGPU
|N10  |  VDDGPU
|N12  |  VDDGPU
|P13  |  VDDGPU
|R12  |  VDDGPU
|[Merged Pins]  F8
|F9  |  VDDIO3
|[Merged Pins]  G8
|G9  |  VDDIO4
|[Merged Pins]  K15
|L14  |  VDDQDDR
|L16  |  VDDQDDR
|M15  |  VDDQDDR
|N14  |  VDDQDDR
|P15  |  VDDQDDR
|R14  |  VDDQDDR
|R16  |  VDDQDDR
|[Merged Pins]  A1
|A22  |  VSS
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[Model Data]
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[End Model Data]
[End Package Model]
|End [Component]
| Models and submodels in the file (84): USB2_HSRX (Input), USB2_HSTX_00_0_01_0011_11 (Output), USB2_HSTX_00_0_10_0101_11 (Output), USB2_HSTX_00_0_11_0111_11 (Output), USB2_HSTX_00_1_01_0011_11 (Output), USB2_HSTX_00_1_10_0101_11 (Output), USB2_HSTX_00_1_11_0111_11 (Output), USB2_HSTX_01_0_01_0011_11 (Output), USB2_HSTX_01_0_10_0101_11 (Output), USB2_HSTX_01_0_11_0111_11 (Output), USB2_HSTX_01_1_01_0011_11 (Output), USB2_HSTX_01_1_10_0101_11 (Output), USB2_HSTX_01_1_11_0111_11 (Output), USB2_HSTX_10_0_01_0011_11 (Output), USB2_HSTX_10_0_10_0101_11 (Output), USB2_HSTX_10_0_11_0111_11 (Output), USB2_HSTX_10_1_01_0011_11 (Output), USB2_HSTX_10_1_10_0101_11 (Output), USB2_HSTX_10_1_11_0111_11 (Output), synopsys_usb3_tx (Output), synopsys_usb3_rx (Input), DPHY_TX_2P5G (Output), DPHY_TX_1P5G (Output), DPHY_RX_1P5G_L1 (Input), DPHY_RX_2P5G_L1 (Input), io8_tt_fs_3v3 (I/O), io8_tt_hs_3v3 (I/O), io8_tt_hslv_fs_1v8 (I/O), io8_tt_hslv_hs_1v8 (I/O), io8_tt_hslv_ls_1v8 (I/O), io8_tt_hslv_ms_1v8 (I/O), io8_tt_i3c_3v3 (I/O_open_drain), io8_tt_ls_3v3 (I/O), io8_tt_ms_3v3 (I/O), isudq_tt_1v8 (Input), isudq_tt_3v3 (Input), mal4drv20_d3_20 (I/O), mal4drv20_d3_24 (I/O), mal4drv20_d3_30 (I/O), mal4drv20_d3_40 (I/O), mal4drv20_d3_60 (I/O), mal4drv20_d4_20 (I/O), mal4drv20_d4_24 (I/O), mal4drv20_d4_30 (I/O), mal4drv20_d4_40 (I/O), mal4drv20_d4_60 (I/O), mal4drv20_dl4_20 (I/O), mal4drv20_dl4_24 (I/O), mal4drv20_dl4_30 (I/O), mal4drv20_dl4_40 (I/O), mal4drv20_dl4_60 (I/O), mal4drv27_d3_28 (I/O), mal4drv27_d3_34 (I/O), mal4drv27_d3_40 (I/O), mal4drv27_d3_53 (I/O), mal4drv27_d3_odt120 (Input), mal4drv27_d3_odt60 (Input), mal4drv27_dl4_28 (I/O), mal4drv27_dl4_34 (I/O), mal4drv27_dl4_40 (I/O), mal4drv27_dl4_53 (I/O), mal4drv27_dl4_odt48 (Input), mal4drv27_dl4_odt60 (Input), mal4drv27_d4_28 (I/O), mal4drv27_d4_34 (I/O), mal4drv27_d4_40 (I/O), mal4drv27_d4_53 (I/O), mal4drv27_d4_odt120 (Input), mal4drv27_d4_odt240 (Input), mal4drv27_d4_odt48 (Input), mal4drv27_d4_odt60 (Input), mal4drv27_d4_odt80 (Input), mal4drv20_d3l_120 (I/O), mal4drv20_d3l_40 (I/O), mal4drv20_d3l_60 (I/O), mal4drv27_d3l_120 (I/O), mal4drv27_d3l_240 (I/O), mal4drv27_d3l_40 (I/O), mal4drv27_d3l_48 (I/O), mal4drv27_d3l_60 (I/O)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
